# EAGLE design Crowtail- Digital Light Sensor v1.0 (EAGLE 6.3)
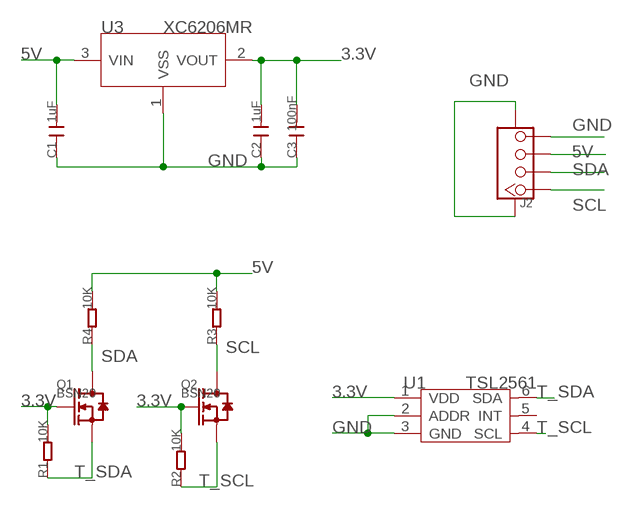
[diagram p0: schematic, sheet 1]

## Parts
C1  1uF  C-0603  [C0603]
C2  1uF  C-0603  [C0603]
C3  100nF  C-0603  [C0603]
J2  TWIG-4P-2.0-SMD-FEMALE-REINFORCE'DD'  [4P-SMD-2.0]
Q1  BSN20  MOSFET-N'SOT23'  [SOT23]
Q2  BSN20  MOSFET-N'SOT23'  [SOT23]
R1  10K  R-0603  [R0603]
R2  10K  R-0603  [R0603]
R3  10K  R-0603  [R0603]
R4  10K  R-0603  [R0603]
U1  TSL2561  TSL2561T  [TMB-6]
U3  XC6206MR  [SOT23]

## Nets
3.3V: C2.2 C3.2 Q1.1(G) Q2.1(G) R1.2 R2.2 U1.1(VDD) U3.2(VOUT)
5V: C1.2 J2.3 R3.2 R4.2 U3.3(VIN)
GND: C1.1 C2.1 C3.1 J2.4 J2.SS1 J2.SS2 U1.2(ADDR) U1.3(GND) U3.1(VSS)
SCL: J2.1 Q2.3(D) R3.1
SDA: J2.2 Q1.3(D) R4.1
T_SCL: Q2.2(S) R2.1 U1.4(SCL)
T_SDA: Q1.2(S) R1.1 U1.6(SDA)
Unconnected: U1.5(INT)

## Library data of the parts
C1-C3 = Discrete:C*: Ceramic Capacitors
J2 = Connector:TWIG-4P-2.0-SMD-FEMALE-REINFORCE
Q1 Q2 = Discrete:MOSFET-N: IRLL014: http://www.vishay.com/docs/91319/sihll014.pdf
R1-R4 = Discrete:R*
U1 = template:TSL2561: Light-TO-Digital Converter
U3 = IC:XC6206: LOW ESR Cap.Compatible Positive Voltage Regulators

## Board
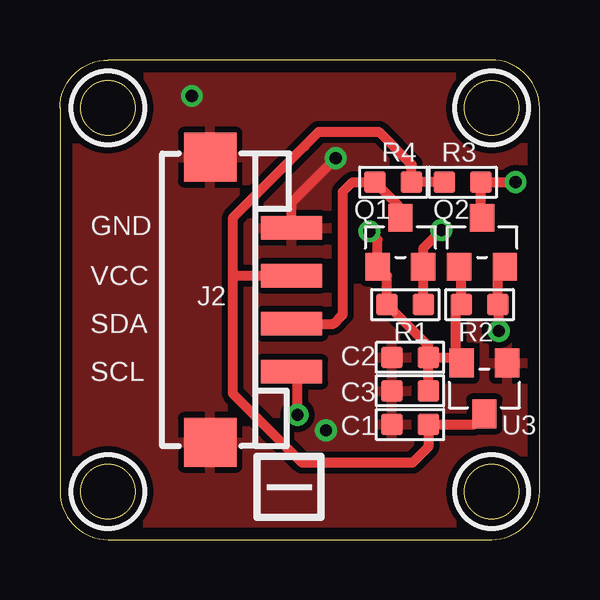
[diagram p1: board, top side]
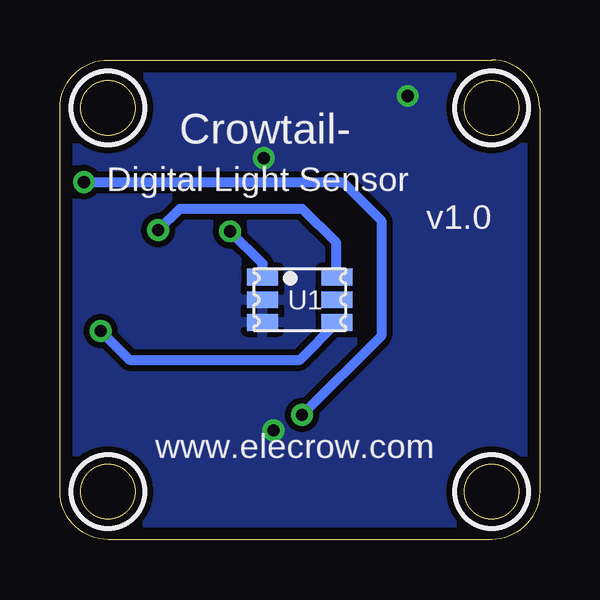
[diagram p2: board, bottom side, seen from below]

Size 20 x 20 mm. Coordinates in mm from the lower left corner, seen from the top.
Outline: 0,18 0,2 arc90 2,0 18,0 arc90 20,2 20,18 arc90 18,20 2,20 arc90 0,18
Outline: circle at 2,18 radius 1.14
Outline: circle at 2,2 radius 1.14
Outline: circle at 18,18 radius 1.14
Outline: circle at 18,2 radius 1.14
Copper layers (1*16): Top 0.035mm / dielectric 1.5mm / Bottom 0.035mm
Design rules "default *": minimum track width 10mil, minimum drill 20mil, track to track 8mil, track to pad 8mil, pad to pad 8mil, via to via 8mil, smd to smd 8mil, copper to edge 20mil, drill to drill 8mil, minimum pad ring 10mil, minimum via ring 8mil, stop-mask expansion 4mil, vias tented up to drill 100mil, thermal gap 10mil
tRestrict: area 0.5,16.5 to 3.5,19.5; area 0.5,0.5 to 3.5,3.5; area 16.5,16.5 to 19.5,19.5; area 16.5,0.5 to 19.5,3.5
bRestrict: area 0.5,16.5 to 3.5,19.5; area 0.5,0.5 to 3.5,3.5; area 16.5,16.5 to 19.5,19.5; area 16.5,0.5 to 19.5,3.5

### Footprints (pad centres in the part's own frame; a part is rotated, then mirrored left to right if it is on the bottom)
C0603 = smd 0.889 x 0.889: 1 -0.762,0; 2 0.762,0
4P-SMD-2.0 = smd 0.965 x 2.54: 1 -3,0; 2 -1,0; 3 1,0; 4 3,0 | smd 2.032 x 2.184: SS1 -5.946,3.4; SS2 5.946,3.4
SOT23 = smd 1.016 x 1.143: 1 -0.95,-1.016; 2 0.95,-1.016; 3 0,1.016
R0603 = smd 0.889 x 0.889: 1 -0.762,0; 2 0.762,0
TMB-6 = smd 1.3 x 0.7: 1 -1.55,0.95; 2 -1.55,0; 3 -1.55,-0.95; 4 1.55,-0.95; 5 1.55,0; 6 1.55,0.95
SOT23' = smd 1.016 x 1.2: 1 -0.95,-1.06; 2 0.95,-1.06; 3 0,1.06

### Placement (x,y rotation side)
C1  14.6,4.8 0 top
C2  14.6,7.6 0 top
C3  14.6,6.2 0 top
J2  9.66,10 90 top
Q1  14.2,12.4 0 top
Q2  17.6,12.4 0 top
R1  14.4,9.8 180 top
R2  17.5,9.8 180 top
R3  16.8,14.9 180 top
R4  13.9,14.9 0 top
U1  10,10 0 bottom
U3  XC6206MR  [SOT23']  17.7,6.3 180 top

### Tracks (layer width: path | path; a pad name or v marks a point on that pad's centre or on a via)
3.3V  (via drill 0.51)
  Top 0.406: Q2.1 16.74,11.3 R2.2 16.51,9.57 16.51,7.6 | C2.2 16.51,7.6 | 16.51,7.6 U3.2 | C3.2 C2.2 | C2.2 15.36,8.08 R1.2 13.64,11 Q1.1 13.25,12.5 v12.9,12.85
  Bottom 0.406: U1.1 11.55,11.5 v12.9,12.85
5V
  Top 0.406: R3.2 R4.2 14.66,15.64 13.3,17 10.8,17 10.2,16.4 | U3.3 17.26,4.8 C1.2 15.36,3.86 14.7,3.2 10.1,3.2 7.2,6.1 7.2,11 | 7.2,13.4 7.2,11 | J2.3 7.2,11 | 7.2,13.4 | 7.2,13.4 10.2,16.4 | 10.2,16.4
GND  (via drill 0.51)
  Top 0.406: J2.4 9.66,14.06 v11.5,15.9
  other vias: 11.1,4.55 5.5,18.5
  pour Bottom (isolate 0.254): -0.51,-0.76 20.45,-0.89 20.32,20.32 -0.64,20.45
  pour Top (isolate 0.254): -0.51,-0.89 20.45,-0.89 20.32,20.45 -0.64,20.45
SCL  (via drill 0.51)
  Top 0.406: Q2.3 17.56,13.42 17.56,14.84 | 17.56,14.84 R3.1 | 17.56,14.84 17.5,14.9 v19,14.9 | v9.9,5.2 9.9,6.9 J2.1
  Bottom 0.406: v19,14.9 8.2,14.9 6.6,13.3 6.6,8.5 v9.9,5.2
SDA
  Top 0.406: R4.1 13.14,14.78 | R4.1 12.2,14.9 11.8,14.5 11.8,9.4 11.4,9 J2.2 | Q1.3 14.08,13.42 14.08,13.95 R4.1
T_SCL  (via drill 0.51)
  Top 0.406: Q2.2 18.26,11.1 R2.1 18.3,9.76 v18.3,8.7
  Bottom 0.406: U1.4 10,7.5 17.1,7.5 v18.3,8.7
T_SDA  (via drill 0.51)
  Top 0.406: R1.1 15.16,11.1 | 15.16,11.1 Q1.2 | 15.16,11.1 15.16,12.16 v15.9,12.9
  Bottom 0.406: U1.6 8.5,11 8.5,12.4 9.9,13.8 15,13.8 v15.9,12.9

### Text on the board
tPlace: GND | VCC | SDA | SCL | I
bPlace: Crowtail- | Digital Light Sensor | v1.0 | www.elecrow.com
